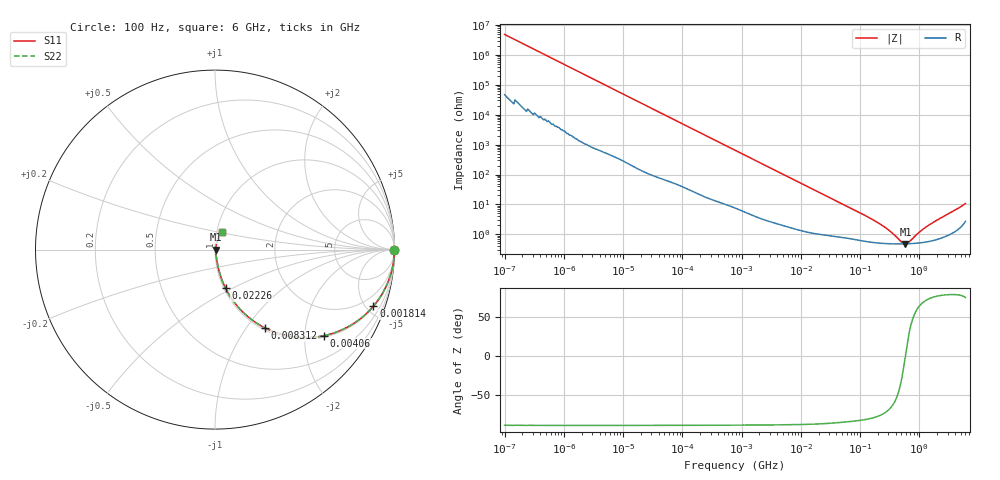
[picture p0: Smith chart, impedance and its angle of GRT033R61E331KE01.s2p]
!Murata Part Number: GRT033R61E331KE01
!These Parameters are Measured in Series Mode Connection
!Data Generated on Jun 19, 2026
!  o--ll--o
!Port1  Port2
!  o------o
!Operation Temp=25[degC], DC Bias Voltage=0[V]
!Freq. Start=100[Hz] Stop=6[GHz] 401[Steps]
# Hz S RI R 50
!Freq.(Hz) S11(Real) S11(Imag) S21(Real) S21(Imag) S12(Real) S12(Imag) S22(Real) S22(Imag)
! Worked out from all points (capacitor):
!   401 points, 100 Hz to 6 GHz, reference 50 ohm
!   read as one part in series: C = 328 pF near 109 Hz
!   lowest |Z| = 481 mohm at 584.8 MHz (marker M1)
!   series resonance near 582.5 MHz, so ESL is about 230 pH
!   S11 on the Smith chart (normalised r, x): 100 Hz: open; 1.814 MHz: 1.08, -5.57; 4.06 MHz: 1.04, -2.50; 8.312 MHz: 1.03, -1.23; 22.26 MHz: 1.02, -0.46; 6 GHz: 1.05, +0.21
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100  1 -2.07e-05  2e-07 2.07e-05  2e-07 2.07e-05  1 -2.07e-05
479  1 -9.84e-05  7e-07 9.84e-05  7e-07 9.84e-05  1 -9.84e-05
2008  1 -0.00041  2.2e-06 0.00041  2.2e-06 0.00041  1 -0.00041
40335  0.9999 -0.00816  0.000118 0.00816  0.000118 0.00816  0.9999 -0.00816
241822  0.9972 -0.0484  0.00276 0.0484  0.00276 0.0484  0.9972 -0.0484
774597  0.975 -0.1502  0.025 0.1502  0.025 0.1502  0.975 -0.1502
1813585  0.8824 -0.3154  0.1176 0.3154  0.1176 0.3154  0.8824 -0.3154
2713602  0.7734 -0.4112  0.2266 0.4112  0.2266 0.4112  0.7734 -0.4112
4060267  0.6081 -0.4794  0.3919 0.4794  0.3919 0.4794  0.6081 -0.4794
5809218  0.436 -0.4857  0.564 0.4857  0.564 0.4857  0.436 -0.4857
8311524  0.2791 -0.4368  0.7209 0.4368  0.7209 0.4368  0.2791 -0.4368
1.555665e7  0.1061 -0.2919  0.8939 0.2919  0.8939 0.2919  0.1061 -0.2919
2.225763e7  0.0591 -0.2156  0.9409 0.2156  0.9409 0.2156  0.0591 -0.2156
4.983056e7  0.0184 -0.1016  0.9816 0.1016  0.9816 0.1016  0.0184 -0.1016
1.334425e8  0.00706 -0.0378  0.9929 0.0378  0.9929 0.0378  0.00706 -0.0378
3.124326e8  0.00496 -0.0123  0.995 0.0123  0.995 0.0123  0.00496 -0.0123
5.112761e8  0.00476 -0.00243  0.9952 0.00243  0.9952 0.00243  0.00476 -0.00243
5.847788e8  0.00478 7.5e-05  0.9952 -7.5e-05  0.9952 -7.5e-05  0.00478 7.5e-05
6.688484e8  0.00483 0.00258  0.9952 -0.00258  0.9952 -0.00258  0.00483 0.00258
1.000774e9  0.00523 0.0105  0.9948 -0.0105  0.9948 -0.0105  0.00523 0.0105
1.431855e9  0.00604 0.0189  0.994 -0.0189  0.994 -0.0189  0.00604 0.0189
6e9  0.0362 0.0971  0.9638 -0.0971  0.9638 -0.0971  0.0362 0.0971
